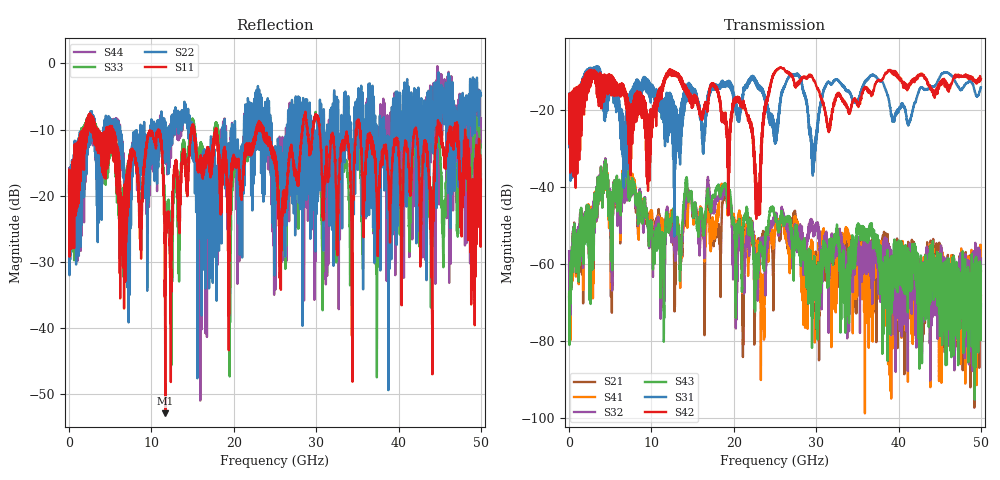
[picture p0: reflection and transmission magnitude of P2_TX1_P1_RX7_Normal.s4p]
!Keysight Technologies,N5225B,MY57041031,A.13.20.10
!Date: Friday, May 31, 2019 11:24:47
!Correction: S11(Full 4 Port(1,2,3,4))
!S12(Full 4 Port(1,2,3,4))
!S13(Full 4 Port(1,2,3,4))
!S14(Full 4 Port(1,2,3,4))
!S21(Full 4 Port(1,2,3,4))
!S22(Full 4 Port(1,2,3,4))
!S23(Full 4 Port(1,2,3,4))
!S24(Full 4 Port(1,2,3,4))
!S31(Full 4 Port(1,2,3,4))
!S32(Full 4 Port(1,2,3,4))
!S33(Full 4 Port(1,2,3,4))
!S34(Full 4 Port(1,2,3,4))
!S41(Full 4 Port(1,2,3,4))
!S42(Full 4 Port(1,2,3,4))
!S43(Full 4 Port(1,2,3,4))
!S44(Full 4 Port(1,2,3,4))
!S4P File: Measurements: <S11,S12,S13,S14>,
!<S21,S22,S23,S24>,
!<S31,S32,S33,S34>,
!<S41,S42,S43,S44>:
# Hz S  dB  R 50.0
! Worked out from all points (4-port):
!   5000 points, 10 MHz to 50 GHz, reference 50 ohm
!   strongest paths, dB at 10 MHz, 12.51 GHz, 25.01 GHz, 37.51 GHz, 50 GHz:
!     S42: -19.6, -9.7, -10.4, -12.3, -12.1
!     S31: -19.5, -17.3, -28.8, -12.1, -14.2
!     S43: -68.5, -47.7, -47.4, -54.9, -70.5
!     S32: -56.7, -51.7, -47.1, -57.5, -58.7
!     S41: -67.8, -46.2, -51.4, -58.8, -68.2
!     S21: -60.6, -49.6, -50.9, -60.7, -62.0
!   lowest |S11| = -52.9 dB at 11.69 GHz (marker M1), VSWR 1.00, Z = 49.8 - j0.116 ohm
!   |S11| at or under -10 dB: 5.36 GHz to 10.81 GHz (5.45 GHz wide, 67.4 % of centre); 17.89 GHz to 22.7 GHz (4.805 GHz wide, 23.7 % of centre); 35.31 GHz to 41.96 GHz (6.646 GHz wide, 17.2 % of centre)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
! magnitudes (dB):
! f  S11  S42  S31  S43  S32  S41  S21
! 10 MHz  -19.6  -19.6  -19.5  -68.5  -56.7  -67.8  -60.6
! 4.35 GHz  -16.2  -16.7  -17.8  -34.4  -33.9  -34.4  -33.9
! 11.69 GHz  -52.9  -11.9  -22.9  -51.7  -52.6  -50.8  -51.5
! 21.14 GHz  -16.7  -19.2  -16.0  -50.4  -57.9  -54.9  -81.0
! 22.93 GHz  -9.7  -40.2  -13.4  -63.8  -68.1  -54.5  -53.7
! 25.47 GHz  -22.2  -9.2  -22.4  -50.7  -50.9  -48.9  -51.0
! 50 GHz  -17.6  -12.1  -14.2  -70.5  -58.7  -68.2  -62.0
